// Version 2.0, 05.09.99: Änderungen:
// Umstrukturierungen und Bearbeitungzeitoptimierung,
// Quittierung von DB71-Aufträgen sofort
// FC90_5

FUNCTION FC 90 : VOID
TITLE = ANSTEUERUNG QUIT_WZV
VERSION : 2.0

BEGIN
NETWORK
TITLE =Quittung Werkzeug beladen beendet Magazin
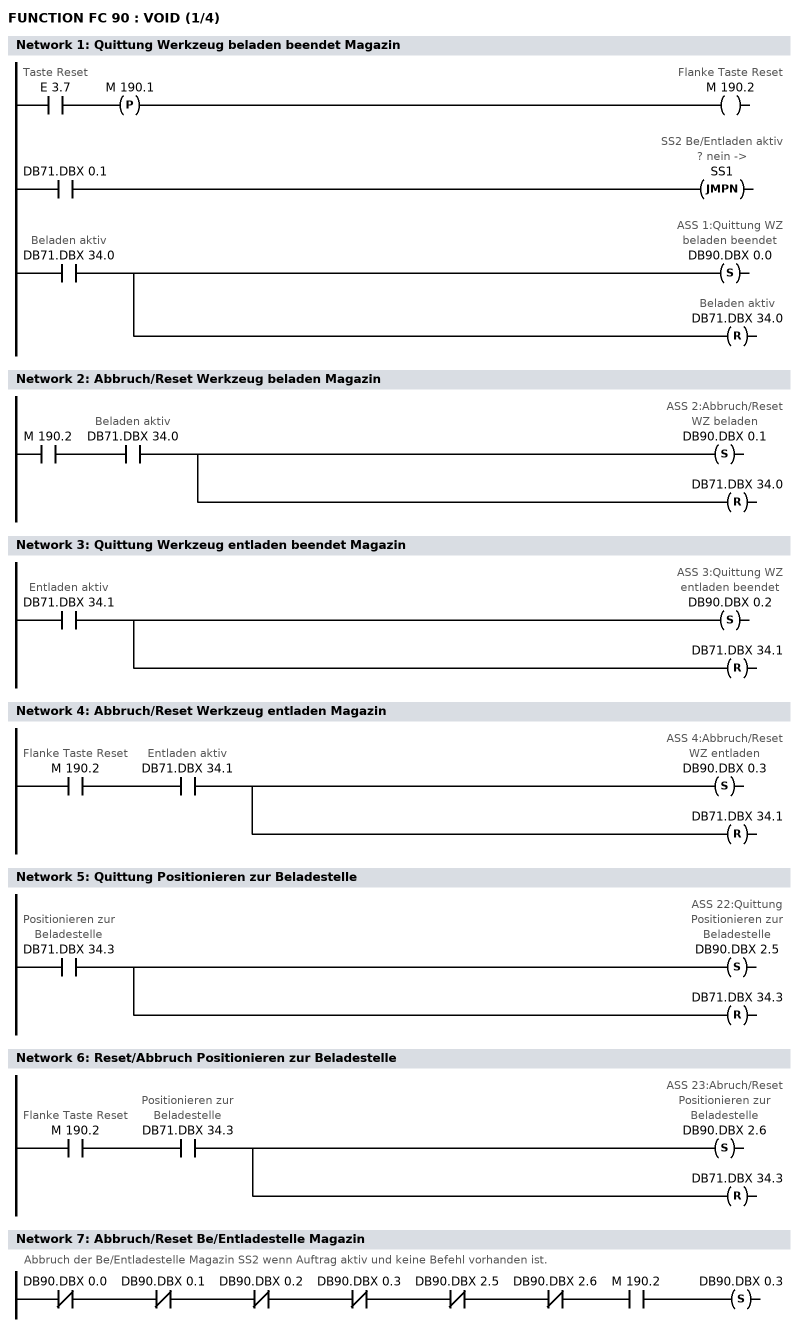
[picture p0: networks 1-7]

      U     E      3.7; // Taste Reset
      FP    M    190.1;
      =     M    190.2; // Flanke Taste Reset
	U	DB71.DBX	0.1;
	SPBN  SS1; // SS2 Be/Entladen aktiv ? nein ->
      U     DB71.DBX   34.0; // Beladen aktiv
//    U     M    190.0; // Flanke beladen Magazin beendet
      S     DB90.DBX    0.0; // ASS 1:Quittung WZ beladen beendet
	R	DB71.DBX   34.0; // Beladen aktiv
NETWORK
TITLE =Abbruch/Reset Werkzeug beladen Magazin

      U     M    190.2;
      U     DB71.DBX   34.0; // Beladen aktiv
      S     DB90.DBX    0.1; // ASS 2:Abbruch/Reset WZ beladen
	R	DB71.DBX   34.0;
NETWORK
TITLE =Quittung Werkzeug entladen beendet Magazin

      U     DB71.DBX   34.1; // Entladen aktiv
//    U     M    190.3; // Flanke entladen Magazin beendet
      S     DB90.DBX    0.2; // ASS 3:Quittung WZ entladen beendet
	R	DB71.DBX	34.1;
NETWORK
TITLE =Abbruch/Reset Werkzeug entladen Magazin

      U     M    190.2; // Flanke Taste Reset
      U     DB71.DBX   34.1; // Entladen aktiv
      S     DB90.DBX    0.3; // ASS 4:Abbruch/Reset WZ entladen
	R	DB71.DBX   34.1;

NETWORK
TITLE =Quittung Positionieren zur Beladestelle

      U     DB71.DBX   34.3;  // Positionieren zur Beladestelle
//    U     M    193.2; // Positionieren beendet
      S     DB90.DBX    2.5; // ASS 22:Quittung Positionieren zur Beladestelle
	R	DB71.DBX   34.3;
NETWORK
TITLE =Reset/Abbruch Positionieren zur Beladestelle

      U     M    190.2; // Flanke Taste Reset
      U     DB71.DBX   34.3; // Positionieren zur Beladestelle
      S     DB90.DBX    2.6; // ASS 23:Abruch/Reset Positionieren zur Beladestelle
	R	DB71.DBX   34.3;
NETWORK
TITLE =Abbruch/Reset Be/Entladestelle Magazin
//Abbruch der Be/Entladestelle Magazin SS2 wenn Auftrag aktiv und keine Befehl vorhanden ist.

      UN    DB90.DBX    0.0;
      UN    DB90.DBX    0.1;
      UN    DB90.DBX    0.2;
	UN	DB90.DBX	0.3;
	UN    DB90.DBX    2.5;
      UN	DB90.DBX	2.6;
      U     M 	190.2;
      S     DB90.DBX    0.3;

NETWORK
TITLE =Quittung Umladen MMC
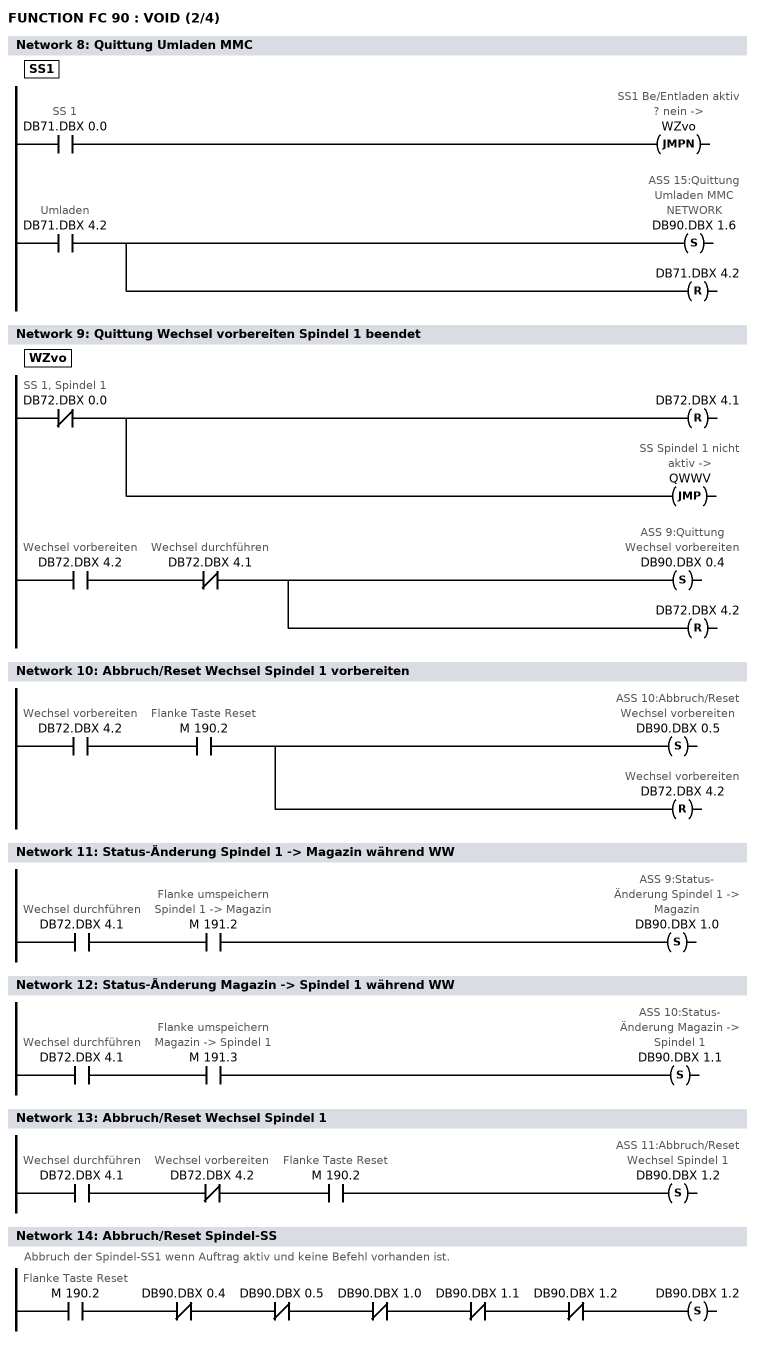
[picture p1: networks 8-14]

SS1:  U     DB71.DBX    0.0; // SS 1
	SPBN  WZvo; // SS1 Be/Entladen aktiv ? nein ->
      U     DB71.DBX    4.2; // Umladen
      S     DB90.DBX    1.6; // ASS 15:Quittung Umladen MMC NETWORK
	R	DB71.DBX	4.2;
NETWORK
TITLE =Quittung Wechsel vorbereiten Spindel 1 beendet

WZvo: UN	DB72.DBX	0.0; // SS 1, Spindel 1
	R	DB72.DBX	4.1;
      SPB  QWWV; // SS Spindel 1 nicht aktiv ->
	U     DB72.DBX    4.2; // Wechsel vorbereiten
      UN    DB72.DBX    4.1; // Wechsel durchführen
//    U     M    190.4; // Flanke Wechsel vorbereitet beendet
      S     DB90.DBX    0.4; // ASS 9:Quittung Wechsel vorbereiten
      R	DB72.DBX	4.2;
NETWORK
TITLE =Abbruch/Reset Wechsel Spindel 1 vorbereiten

      U     DB72.DBX    4.2; // Wechsel vorbereiten
      U     M    190.2; // Flanke Taste Reset
      S     DB90.DBX    0.5; // ASS 10:Abbruch/Reset Wechsel vorbereiten
      R     DB72.DBX    4.2; // Wechsel vorbereiten
NETWORK
TITLE =Status-Änderung Spindel 1 -> Magazin während WW

      U     DB72.DBX    4.1; // Wechsel durchführen
      U     M    191.2; // Flanke umspeichern Spindel 1 -> Magazin
      S     DB90.DBX    1.0; // ASS 9:Status-Änderung Spindel 1 -> Magazin
NETWORK
TITLE =Status-Änderung Magazin -> Spindel 1 während WW

      U     DB72.DBX    4.1; // Wechsel durchführen
      U     M    191.3; // Flanke umspeichern Magazin -> Spindel 1
      S     DB90.DBX    1.1; // ASS 10:Status-Änderung Magazin -> Spindel 1
NETWORK
TITLE =Abbruch/Reset Wechsel Spindel 1

      U     DB72.DBX    4.1; // Wechsel durchführen
      UN    DB72.DBX    4.2; // Wechsel vorbereiten
      U     M    190.2; // Flanke Taste Reset
      S     DB90.DBX    1.2; // ASS 11:Abbruch/Reset Wechsel Spindel 1
NETWORK
TITLE =Abbruch/Reset Spindel-SS
//Abbruch der Spindel-SS1 wenn Auftrag aktiv und keine Befehl vorhanden ist.

	U	M 	190.2; // Flanke Taste Reset
	UN	DB90.DBX	0.4;
      UN    DB90.DBX    0.5;
	UN	DB90.DBX	1.0;
	UN	DB90.DBX	1.1;
      UN    DB90.DBX    1.2;
      S     DB90.DBX    1.2;

NETWORK
TITLE =Quittung Wechsel vorbereiten Spindel 2 beendet
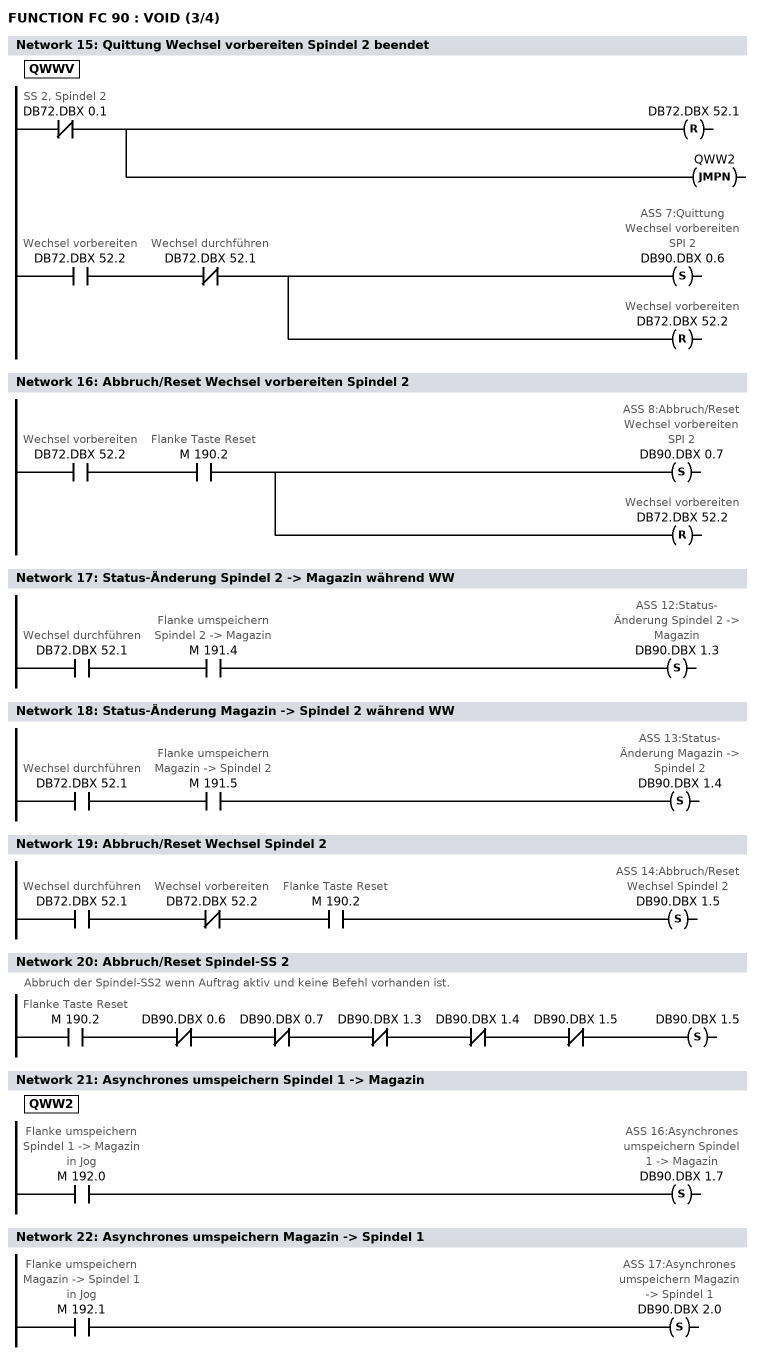
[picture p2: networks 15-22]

QWWV: UN    DB72.DBX    0.1; // SS 2, Spindel 2
      R	DB72.DBX 	52.1;
	SPBN  QWW2;
 	U     DB72.DBX   52.2; // Wechsel vorbereiten
      UN    DB72.DBX   52.1; // Wechsel durchführen
//   U     M    190.7; // Flanke Wechsel vorbereitet Spi 2 beendet
      S     DB90.DBX    0.6; // ASS 7:Quittung Wechsel vorbereiten SPI 2
      R     DB72.DBX   52.2; // Wechsel vorbereiten

NETWORK
TITLE =Abbruch/Reset Wechsel vorbereiten Spindel 2

      U     DB72.DBX   52.2; // Wechsel vorbereiten
      U     M    190.2; // Flanke Taste Reset
      S     DB90.DBX    0.7; // ASS 8:Abbruch/Reset Wechsel vorbereiten SPI 2
      R     DB72.DBX   52.2; // Wechsel vorbereiten
NETWORK
TITLE =Status-Änderung Spindel 2 -> Magazin während WW

      U     DB72.DBX   52.1; // Wechsel durchführen
      U     M    191.4; // Flanke umspeichern Spindel 2 -> Magazin
      S     DB90.DBX    1.3; // ASS 12:Status-Änderung Spindel 2 -> Magazin
NETWORK
TITLE =Status-Änderung Magazin -> Spindel 2 während WW

      U     DB72.DBX   52.1; // Wechsel durchführen
      U     M    191.5; // Flanke umspeichern Magazin -> Spindel 2
      S     DB90.DBX    1.4; // ASS 13:Status-Änderung Magazin -> Spindel 2
NETWORK
TITLE =Abbruch/Reset Wechsel Spindel 2

      U     DB72.DBX   52.1; // Wechsel durchführen
      UN    DB72.DBX   52.2; // Wechsel vorbereiten
      U     M    190.2; // Flanke Taste Reset
      S     DB90.DBX    1.5; // ASS 14:Abbruch/Reset Wechsel Spindel 2
NETWORK
TITLE =Abbruch/Reset Spindel-SS 2
//Abbruch der Spindel-SS2 wenn Auftrag aktiv und keine Befehl vorhanden ist.

	U	M 	190.2; // Flanke Taste Reset
	UN	DB90.DBX	0.6;
      UN    DB90.DBX    0.7;
	UN	DB90.DBX	1.3;
      UN    DB90.DBX    1.4;
      UN    DB90.DBX    1.5;
      S     DB90.DBX    1.5;

NETWORK
TITLE =Asynchrones umspeichern Spindel 1 -> Magazin

QWW2: U     M    192.0; // Flanke umspeichern Spindel 1 -> Magazin in Jog
      S     DB90.DBX    1.7; // ASS 16:Asynchrones umspeichern Spindel 1 -> Magazin
NETWORK
TITLE =Asynchrones umspeichern Magazin -> Spindel 1

      U     M    192.1; // Flanke umspeichern Magazin -> Spindel 1 in Jog
      S     DB90.DBX    2.0; // ASS 17:Asynchrones umspeichern Magazin -> Spindel 1
NETWORK
TITLE =Asynchrones umspeichern Spindel 2 -> Magazin
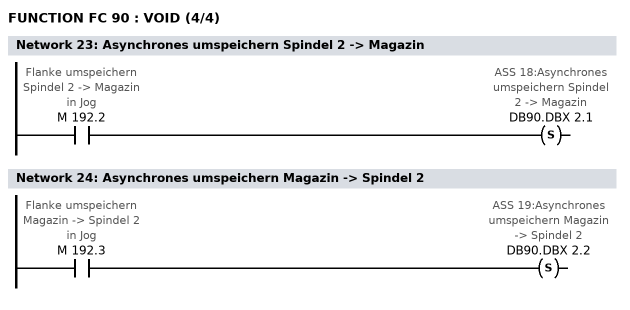
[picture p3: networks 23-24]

      U     M    192.2; // Flanke umspeichern Spindel 2 -> Magazin in Jog
      S     DB90.DBX    2.1; // ASS 18:Asynchrones umspeichern Spindel 2 -> Magazin
NETWORK
TITLE =Asynchrones umspeichern Magazin -> Spindel 2

      U     M    192.3; // Flanke umspeichern Magazin -> Spindel 2 in Jog
      S     DB90.DBX    2.2; // ASS 19:Asynchrones umspeichern Magazin -> Spindel 2
NETWORK
TITLE =Änderung Istposition
// In MW180 steht die aktuelle Istposition der Wechselstelle in Format Int (ist
// vom Anwender zu versorgen).
      L     DB90.DBW   10; // Istposition alt
      L     MW   180; // Istposition neu
      T     DB90.DBW   10;
      <>I   ;
      S     DB90.DBX    2.3; // ASS 20: Änderung Istposition Magazin
NETWORK
TITLE =Fehlerbit löschen

      U     M    192.7; // Taste Fehler löschen
      R     DB90.DBX    4.0; // Fehler Quittung FC 8
NETWORK
TITLE =Aufruf FB 90
// Aufruf nur wenn QUIT_1 (FB90, DB90) bereits übersetzt wurde.
      CALL FB    90 , DB    90 ;

END_FUNCTION

